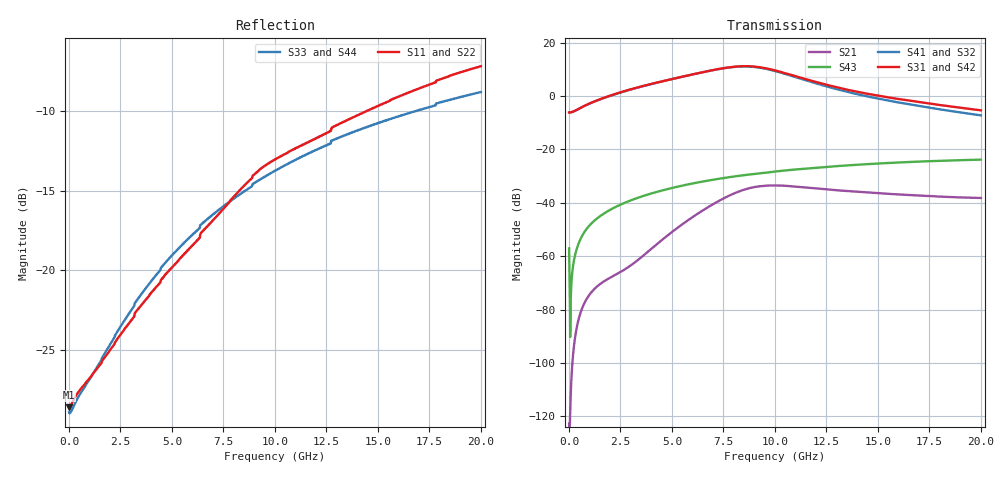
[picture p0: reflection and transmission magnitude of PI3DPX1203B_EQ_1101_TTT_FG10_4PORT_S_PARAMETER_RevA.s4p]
! NPort=4 DATA=2000 NOISE=0 GROUPDELAY=0 COMPLEX_DATAFORMAT=POLAR
! NumOfBlock=1 NumOfParam=0
! .MODEL Smodel S TSTONEFILE=PI3DPX1203B_EQ_1101_TTT_FG10_4PORT_S_PARAMETER_RevA.s4p TYPE=S
!  -- The above .MODEL line can be used for the S element in the netlist.
! The s parameter is extracted from the linear redriver, it is not bi-directional; only s(4,1)s(4,2) and s(3,1)s(3,2)
! should be the insertion loss
!Port definition:
!Port1 = input+
!Port2 = input-
!Port3 = output+
!Port4 = output-
# Hz S MA R  50
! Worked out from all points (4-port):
!   2000 points, 10 MHz to 20 GHz, reference 50 ohm
!   strongest paths, dB at 10 MHz, 5.01 GHz, 10.01 GHz, 15.01 GHz, 20 GHz:
!     S31: -6.2, 6.4, 9.6, 0.1, -5.4
!     S42: -6.2, 6.4, 9.6, 0.1, -5.4
!     S41: -6.2, 6.3, 9.3, -1.0, -7.3
!     S32: -6.2, 6.3, 9.3, -1.0, -7.3
!     S43: -57.1, -34.4, -28.3, -25.3, -23.8
!     S21: -122.7, -50.9, -33.5, -36.4, -38.2
!   lowest |S11| = -28.6 dB at 10 MHz (marker M1), VSWR 1.08, Z = 46.4 - j0.0306 ohm
!   |S11| at or under -10 dB: start of sweep to 14.42 GHz
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1e7  0.03701 -179.5  7.338e-07 10.7  0 0.0  0 0.0
     7.338e-07 10.7  0.03701 -179.5  0 0.0  0 0.0
     0.4917 0.0  0.4917 -180.0  0.03566 178.2  0.001403 -77.8
     0.4917 -180.0  0.4917 0.0  0.001403 -77.8  0.03566 178.2
3.03e9  0.06952 -127.3  0.0006844 144.6  1.326e-10 57.2  2.358e-09 107.8
        0.0006841 144.6  0.06952 -127.3  2.358e-09 107.8  1.326e-10 57.2
        1.342 4.0  1.33 -174.9  0.07492 -126.9  0.0112 77.9
        1.331 -174.9  1.342 4.0  0.0112 77.9  0.07492 -126.9
5.72e9  0.1144 -111.1  0.004537 155.2  1.092e-08 -122.2  1.016e-07 70.3
        0.004537 155.3  0.1144 -111.1  1.016e-07 70.3  1.093e-08 -122.2
        2.397 -38.4  2.395 143.0  0.1242 -117.4  0.02184 66.5
        2.396 143.0  2.397 -38.4  0.02184 66.5  0.1242 -117.4
8.12e9  0.1737 -104.9  0.01555 111.3  2.858e-07 155.6  8.036e-07 21.0
        0.01555 111.3  0.1737 -104.9  8.029e-07 21.0  2.86e-07 155.6
        3.554 -98.3  3.522 82.9  0.1701 -115.8  0.03148 54.3
        3.523 82.9  3.553 -98.3  0.03148 54.3  0.1701 -115.8
9.69e9  0.2168 -107.2  0.02106 67.4  1.021e-06 94.5  1.73e-06 -16.7
        0.02104 67.4  0.2168 -107.2  1.728e-06 -16.7  1.021e-06 94.5
        3.219 -148.9  3.145 32.1  0.2001 -116.1  0.03737 46.0
        3.146 32.1  3.218 -148.9  0.03737 46.0  0.2001 -116.1
1.193e10  0.2586 -109.4  0.01876 26.5  2.789e-06 29.7  3.451e-06 -45.1
          0.01874 26.6  0.2586 -109.3  3.451e-06 -45.0  2.791e-06 29.7
          1.856 162.4  1.75 -16.4  0.2376 -117.4  0.04524 34.6
          1.752 -16.4  1.855 162.4  0.04524 34.6  0.2376 -117.4
2e10  0.4389 -117.7  0.01226 -17.9  2.242e-05 -109.6  3.118e-05 -133.7
      0.01232 -17.6  0.439 -117.7  3.125e-05 -133.7  2.245e-05 -109.6
      0.5382 73.6  0.4339 -94.4  0.3637 -123.9  0.06431 -7.1
      0.4338 -94.5  0.5389 73.6  0.06431 -7.1  0.3637 -123.9
